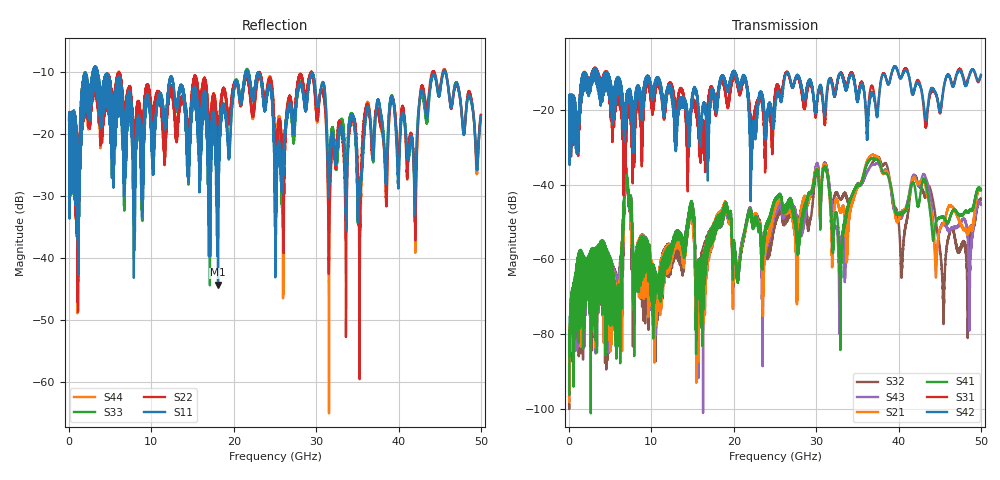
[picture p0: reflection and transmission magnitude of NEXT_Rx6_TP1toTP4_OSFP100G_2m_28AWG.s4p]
! Touchstone data
! Created: 27-Feb-2019 by IdEM 12 (12.1.0)
! COMMENTS
!  Created Wed Feb 27 12:03:36 2019
!  64 Port Network Data from SP1.SP block
!  freq  magS1_1  angS1_1  magS1_2  angS1_2  magS1_3  angS1_3  magS1_4  angS1_4
!  magS1_5  angS1_5  magS1_6  angS1_6  magS1_7  angS1_7  magS1_8  angS1_8
!  magS1_9  angS1_9  magS1_10  angS1_10  magS1_11  angS1_11  magS1_12  angS1_12
!  magS1_13  angS1_13  magS1_14  angS1_14  magS1_15  angS1_15  magS1_16  angS1_16
!  magS1_17  angS1_17  magS1_18  angS1_18  magS1_19  angS1_19  magS1_20  angS1_20
!  magS1_21  angS1_21  magS1_22  angS1_22  magS1_23  angS1_23  magS1_24  angS1_24
!  magS1_25  angS1_25  magS1_26  angS1_26  magS1_27  angS1_27  magS1_28  angS1_28
!  magS1_29  angS1_29  magS1_30  angS1_30  magS1_31  angS1_31  magS1_32  angS1_32
!  magS1_33  angS1_33  magS1_34  angS1_34  magS1_35  angS1_35  magS1_36  angS1_36
!  magS1_37  angS1_37  magS1_38  angS1_38  magS1_39  angS1_39  magS1_40  angS1_40
!  magS1_41  angS1_41  magS1_42  angS1_42  magS1_43  angS1_43  magS1_44  angS1_44
!  magS1_45  angS1_45  magS1_46  angS1_46  magS1_47  angS1_47  magS1_48  angS1_48
!  magS1_49  angS1_49  magS1_50  angS1_50  magS1_51  angS1_51  magS1_52  angS1_52
!  magS1_53  angS1_53  magS1_54  angS1_54  magS1_55  angS1_55  magS1_56  angS1_56
!  magS1_57  angS1_57  magS1_58  angS1_58  magS1_59  angS1_59  magS1_60  angS1_60
!  magS1_61  angS1_61  magS1_62  angS1_62  magS1_63  angS1_63  magS1_64  angS1_64
!  magS2_1  angS2_1  magS2_2  angS2_2  magS2_3  angS2_3  magS2_4  angS2_4
!  magS2_5  angS2_5  magS2_6  angS2_6  magS2_7  angS2_7  magS2_8  angS2_8
!  magS2_9  angS2_9  magS2_10  angS2_10  magS2_11  angS2_11  magS2_12  angS2_12
!  magS2_13  angS2_13  magS2_14  angS2_14  magS2_15  angS2_15  magS2_16  angS2_16
!  magS2_17  angS2_17  magS2_18  angS2_18  magS2_19  angS2_19  magS2_20  angS2_20
!  magS2_21  angS2_21  magS2_22  angS2_22  magS2_23  angS2_23  magS2_24  angS2_24
!  magS2_25  angS2_25  magS2_26  angS2_26  magS2_27  angS2_27  magS2_28  angS2_28
!  magS2_29  angS2_29  magS2_30  angS2_30  magS2_31  angS2_31  magS2_32  angS2_32
!  magS2_33  angS2_33  magS2_34  angS2_34  magS2_35  angS2_35  magS2_36  angS2_36
!  magS2_37  angS2_37  magS2_38  angS2_38  magS2_39  angS2_39  magS2_40  angS2_40
!  magS2_41  angS2_41  magS2_42  angS2_42  magS2_43  angS2_43  magS2_44  angS2_44
!  magS2_45  angS2_45  magS2_46  angS2_46  magS2_47  angS2_47  magS2_48  angS2_48
!  magS2_49  angS2_49  magS2_50  angS2_50  magS2_51  angS2_51  magS2_52  angS2_52
!  magS2_53  angS2_53  magS2_54  angS2_54  magS2_55  angS2_55  magS2_56  angS2_56
!  magS2_57  angS2_57  magS2_58  angS2_58  magS2_59  angS2_59  magS2_60  angS2_60
!  magS2_61  angS2_61  magS2_62  angS2_62  magS2_63  angS2_63  magS2_64  angS2_64
!  magS3_1  angS3_1  magS3_2  angS3_2  magS3_3  angS3_3  magS3_4  angS3_4
!  magS3_5  angS3_5  magS3_6  angS3_6  magS3_7  angS3_7  magS3_8  angS3_8
!  magS3_9  angS3_9  magS3_10  angS3_10  magS3_11  angS3_11  magS3_12  angS3_12
!  magS3_13  angS3_13  magS3_14  angS3_14  magS3_15  angS3_15  magS3_16  angS3_16
!  magS3_17  angS3_17  magS3_18  angS3_18  magS3_19  angS3_19  magS3_20  angS3_20
!  magS3_21  angS3_21  magS3_22  angS3_22  magS3_23  angS3_23  magS3_24  angS3_24
!  magS3_25  angS3_25  magS3_26  angS3_26  magS3_27  angS3_27  magS3_28  angS3_28
!  magS3_29  angS3_29  magS3_30  angS3_30  magS3_31  angS3_31  magS3_32  angS3_32
!  magS3_33  angS3_33  magS3_34  angS3_34  magS3_35  angS3_35  magS3_36  angS3_36
!  magS3_37  angS3_37  magS3_38  angS3_38  magS3_39  angS3_39  magS3_40  angS3_40
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# Hz S MA R 50
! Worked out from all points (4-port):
!   5000 points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, 10 MHz to 50 GHz, reference 50 ohm
!   strongest paths, dB at 10 MHz, 12.51 GHz, 25.01 GHz, 37.51 GHz, 50 GHz:
!     S42: -18.1, -16.3, -19.6, -20.0, -10.7
!     S31: -18.0, -14.0, -15.8, -18.9, -11.0
!     S41: -95.5, -56.2, -43.8, -33.5, -41.4
!     S21: -97.8, -56.6, -45.9, -32.7, -41.5
!     S43: -96.7, -56.8, -47.3, -34.2, -45.4
!     S32: -99.0, -57.2, -49.7, -32.7, -43.8
!   lowest |S11| = -44.3 dB at 18.09 GHz (marker M1), VSWR 1.01, Z = 49.5 + j0.362 ohm
!   |S11| at or under -10 dB: 3.49 GHz to 21.47 GHz (17.98 GHz wide, 144 % of centre); 21.77 GHz to 45.47 GHz (23.7 GHz wide, 70.5 % of centre); 45.66 GHz to end of sweep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
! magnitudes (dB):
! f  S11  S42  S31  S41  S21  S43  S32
! 10 MHz  -17.7  -18.1  -18.0  -95.5  -97.8  -96.7  -99.0
! 5.96 GHz  -15.6  -15.5  -17.7  -78.3  -71.8  -66.1  -65.4
! 6.94 GHz  -23.9  -20.4  -28.7  -37.4  -38.0  -39.1  -39.8
! 10.58 GHz  -16.5  -12.3  -14.2  -64.3  -65.8  -66.5  -65.6
! 18.09 GHz  -44.3  -16.9  -16.7  -49.6  -48.5  -49.4  -48.3
! 45.44 GHz  -10.1  -14.7  -14.9  -48.6  -50.6  -50.7  -72.3
! 50 GHz  -17.2  -10.7  -11.0  -41.4  -41.5  -45.4  -43.8
